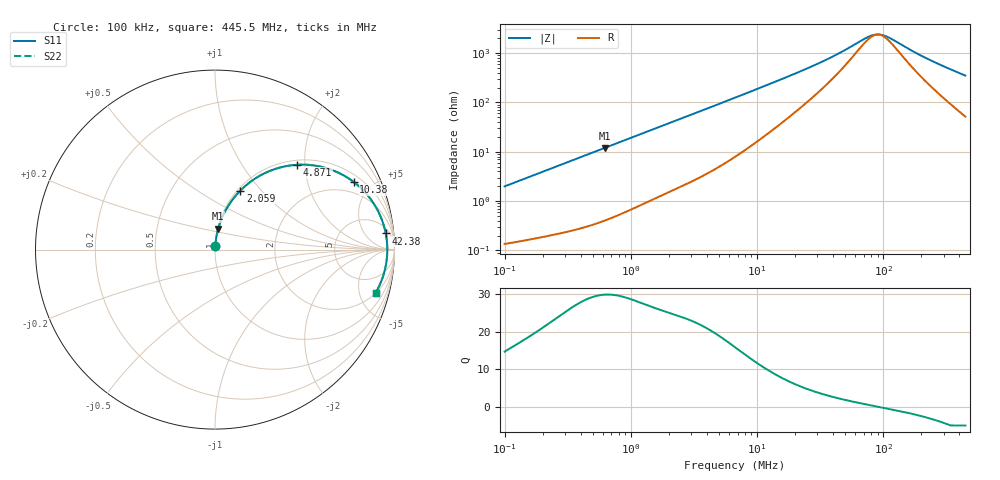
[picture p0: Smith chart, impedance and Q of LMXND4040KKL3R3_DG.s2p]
! LMXND4040KKL3R3_DG  S-PARAMETER MODEL  ( General Type )
! Model Generated by TAIYO YUDEN Corporation (https://www.yuden.co.jp/en/)
! Version 1.0
! TAIYO YUDEN Control No. 191023NI43SB-FBB
! Copyright(c) 2019 TAIYO YUDEN CO.,LTD. All Rights Reserved.
! Product Description (link to TY-COMPAS)
! https://ds.yuden.co.jp/TYCOMPAS/or/detail?pn=LMXND4040KKL3R3MDG&u=M
! Products Name : Inductors
! Characteristics :
!  Inductance : 3.3 uH , SRF(min) : 58 MHz , DC Resistance(max) : 0.12 Ohm
!  Rated Current : Saturation :1100 mA , Temp Rise : 1400 mA (40 degC)
!  Case Size : 4.0 x 4.0 / 0.157 x 0.157 [mm/inch] , Thickness : 1 / 0.039 [mm/inch]
!  (Conditions: Temperature = 25 degC , DC Bias Current/Voltage = 0A / 0V)
! External Node Assignments :
!  1  o---GGG---o  2
! GND o---------o GND
! Frequency Range : 0.1MHz  -  445.549718MHz  [ 402 STEP ]
# MHz S RI R 50
! Freq[MHz].  S11 Real  S11 Imag  S21 Real  S21 Imag  S12 Real  S12 Imag  S22 Real  S22 Imag
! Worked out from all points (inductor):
!   401 points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, 100 kHz to 445.5 MHz, reference 50 ohm
!   read as one part in series: L = 3.14 uH near 104.3 kHz
!   highest Q = 29.8 at 621.8 kHz (marker M1), where L = 3.07 uH
!   self-resonance near 90.24 MHz
!   S11 on the Smith chart (normalised r, x): 100 kHz: 1.00, +0.04; 2.059 MHz: 1.03, +0.78; 4.871 MHz: 1.10, +1.82; 10.38 MHz: 1.35, +3.89; 42.38 MHz: 8, +17; 445.5 MHz: 2.03, -6.94
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0.1  0.00174 0.0197  0.9983 -0.0197  0.9983 -0.0197  0.00174 0.0197
0.217532  0.00374 0.0423  0.9963 -0.0423  0.9963 -0.0423  0.00374 0.0423
0.408498  0.009 0.0782  0.991 -0.0782  0.991 -0.0782  0.009 0.0782
0.621777  0.018 0.1173  0.982 -0.1173  0.982 -0.1173  0.018 0.1173
1.073527  0.0469 0.1944  0.9531 -0.1944  0.9531 -0.1944  0.0469 0.1944
1.668708  0.1002 0.2815  0.8998 -0.2815  0.8998 -0.2815  0.1002 0.2815
2.058745  0.1414 0.3289  0.8586 -0.3289  0.8586 -0.3289  0.1414 0.3289
3.068493  0.2588 0.4166  0.7412 -0.4166  0.7412 -0.4166  0.2588 0.4166
3.948136  0.3603 0.4569  0.6397 -0.4569  0.6397 -0.4569  0.3603 0.4569
4.870959  0.4564 0.4726  0.5436 -0.4726  0.5436 -0.4726  0.4564 0.4726
6.81664  0.6127 0.4562  0.3873 -0.4562  0.3873 -0.4562  0.6127 0.4562
10.37565  0.7724 0.3771  0.2276 -0.3771  0.2276 -0.3771  0.7724 0.3771
16.12806  0.875 0.2704  0.125 -0.2704  0.125 -0.2704  0.875 0.2704
27.26705  0.932 0.1601  0.068 -0.1601  0.068 -0.1601  0.932 0.1601
42.38432  0.9512 0.0902  0.0488 -0.0902  0.0488 -0.0902  0.9512 0.0902
70.16799  0.9591 0.0279  0.0409 -0.0279  0.0409 -0.0279  0.9591 0.0279
81.28206  0.9598 0.0115  0.0402 -0.0115  0.0402 -0.0115  0.9598 0.0115
94.15652  0.9599 -0.00466  0.0401 0.00466  0.0401 0.00466  0.9599 -0.00466
111.3854  0.9594 -0.0233  0.0406 0.0233  0.0406 0.0233  0.9594 -0.0233
218.1424  0.9476 -0.1085  0.0524 0.1085  0.0524 0.1085  0.9476 -0.1085
318.376  0.9281 -0.1721  0.0719 0.1721  0.0719 0.1721  0.9281 -0.1721
445.5497  0.8944 -0.242  0.1056 0.242  0.1056 0.242  0.8944 -0.242
